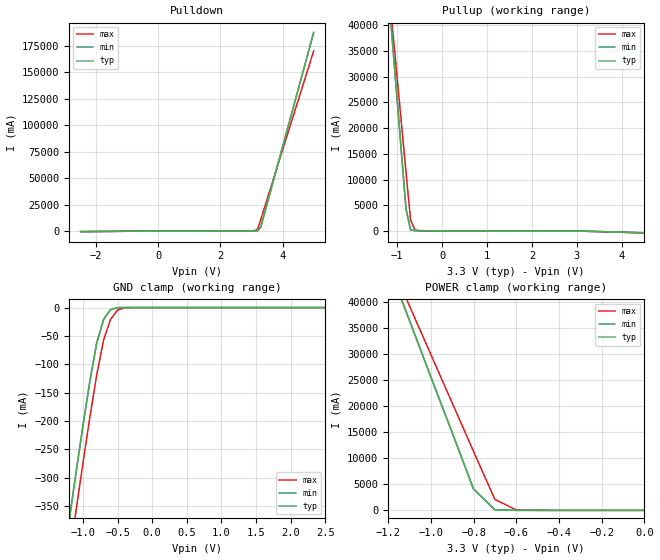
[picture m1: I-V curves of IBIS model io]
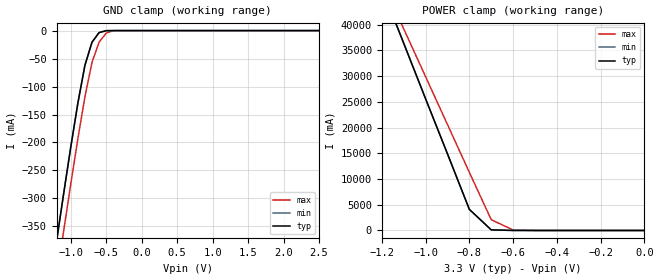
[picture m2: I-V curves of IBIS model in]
[IBIS Ver]   1.1
[File name]   m69737tq.ibs
[File Rev]   1.0
[Date]   4/7/98
[Source]   This file originated at Motorola FSRAM.
[Notes]
 1. This I/O model good for MCM69737 128Kx36 4Meg BurstRAM "F" and "P"
 versions (TQFP).
[Disclaimer]   Data is for modeling purposes only and is not guaranteed
[Component]   128Kx36 4M BurstRAM
[Manufacturer] Motorola
[Package]
|  RLC Data is subject to change after further study of package
|		typ		min		max
R_pkg		200m		150m		250m
L_pkg		5.5nH		4nH		7nH
C_pkg		2pF		1.5pF		2.5pF
[Pin]		signal_name	model_name	R_pin		L_pin		C_pin
1		DCc		io		NA		NA		NA
2		DCc		io		NA		NA		NA
3		DCc		io		NA		NA		NA
4		VDDQ		POWER		NA		NA		NA
5		VSS		GND		NA		NA		NA
6		DCc		io		NA		NA		NA
7		DCc		io		NA		NA		NA
8		DQc		io		NA		NA		NA
9		DQc		io		NA		NA		NA
10		VSS		GND		NA		NA		NA
11		VDDQ		POWER		NA		NA		NA
12		DQc		io		NA		NA		NA
13		DQc		io		NA		NA		NA
14		NC		NC		NA		NA		NA
15		VDD		POWER		NA		NA		NA
16		NC		NC		NA		NA		NA
17		VSS		GND		NA		NA		NA
18		DQd		io		NA		NA		NA
19		DQd	 	io		NA		NA		NA
20		VDDQ		POWER		NA		NA		NA
21		VSS		GND		NA		NA		NA
22		DQd		io		NA		NA		NA
23		DQd		io		NA		NA		NA
24		DQd		io		NA		NA		NA
25		DCd		NC		NA		NA		NA
26		VSS		GND		NA		NA		NA
27		VDDQ		POWER		NA		NA		NA
28		DCd		io		NA		NA		NA
29		DCd		io		NA		NA		NA
30		DCd		io		NA		NA		NA
31		LBO#		NC		NA		NA		NA
32		SA		in		NA		NA		NA
33		SA		in		NA		NA		NA
34		SA		in		NA		NA		NA
35		SA		in		NA		NA		NA
36		SA1		in		NA		NA		NA
37		SA0		in		NA		NA		NA
38		NC		NC		NA		NA		NA
39		NC		NC		NA		NA		NA
40		VSS		GND		NA		NA		NA
41		VDD		POWER		NA		NA		NA
42		NC		NC		NA		NA		NA
43		NC		NC		NA		NA		NA
44		SA		in		NA		NA		NA
45		SA		in		NA		NA		NA
46		SA		in		NA		NA		NA
47		SA		in		NA		NA		NA
48		SA		in		NA		NA		NA
49		SA		in		NA		NA		NA
50		SA		in		NA		NA		NA
51		DQa		io		NA		NA		NA
52		DQa		io		NA		NA		NA
53		DQa		io		NA		NA		NA
54		VDDQ		POWER		NA		NA		NA
55		VSS		GND		NA		NA		NA
56		DQa		io		NA		NA		NA
57		DQa		io		NA		NA		NA
58		DQa		io		NA		NA		NA
59		DQa		io		NA		NA		NA
60		VSS		GND		NA		NA		NA
61		VDDQ		POWER		NA		NA		NA
62		DQa		io		NA		NA		NA
63		DQa		io		NA		NA		NA
64		NC		NC		NA		NA		NA
65		VDD		POWER		NA		NA		NA
66		NC		NC		NA		NA		NA
67		VSS		GND		NA		NA		NA
68		DQb		io		NA		NA		NA
69		DQb		io		NA		NA		NA
70		VDDQ		POWER		NA		NA		NA
71		VSS		GND		NA		NA		NA
72		DQb		io		NA		NA		NA
73		DQb		io		NA		NA		NA
74		DQb		io		NA		NA		NA
75		DQb		io		NA		NA		NA
76		VSS		GND		NA		NA		NA
77		VDDQ		POWER		NA		NA		NA
78		DQb		io		NA		NA		NA
79		DQb		io		NA		NA		NA
80		DQb		io		NA		NA		NA
81		SA		in		NA		NA		NA
82		SA		in		NA		NA		NA
83		ADV		in		NA		NA		NA
84		ADSP		in		NA		NA		NA
85		ADSC		in		NA		NA		NA
86		G		in		NA		NA		NA
87		SW		in		NA		NA		NA
88		SGW		in		NA		NA		NA
89		K		in		NA		NA		NA
90		VSS		GND		NA		NA		NA
91		VDD		POWER		NA		NA		NA
92		SE3		in		NA		NA		NA
93		SBA		in		NA		NA		NA
94		SBB		in		NA		NA		NA
95		NC		NC		NA		NA		NA
96		NC		NC		NA		NA		NA
97		SE2		in		NA		NA		NA
98		SE1		in		NA		NA		NA
99		SA		in		NA		NA		NA
100		SA		in		NA		NA		NA
| Models and submodels in the file (2): io (I/O), in (Input)
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| BI-DIRECTIONAL I/O MODEL
[Model]   io
Model_type  I/O
Polarity   Non-Inverting
Enable   Active-Low
|signals  DQa, DQb, DQc, DQd
|Variable   typ   min   max
C_comp   7pF   NA   8pF
|Variable   typ   min   max
[Voltage range]   3.3   3.1  3.6
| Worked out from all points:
|   slope of the pulldown table from 0 to 0.495 V, typ, clamps not added: 19.4 ohm
|   slope of the pullup table from 0 to 0.495 V, typ, clamps not added: 18.1 ohm
|   GND clamp passes 1 mA (typ) near -0.52 V on its own axis
|   POWER clamp passes 1 mA (typ) near -0.53 V on its own axis
|Temp used   50C   100C   0C
|Variable   typ   min   max
|NOTE: All V/I tables should have at least 3 entries.
|   0.0 volts, 2*supply_voltage and -supply_voltage
[Pulldown]
|Voltage	Typical			Minimum		Maximum
-2.5V     -454.1mA   -454.2mA   -476.2mA
3V        59.2mA     68.8mA     53.1mA
3.1V      62.5mA     72.1mA     142.5mA
3.2V      178.6mA    188.2mA    2.1A
3.3V      4.2A       4.2A       11.3A
5V        187.4A     187.4A     170A
[Pullup]
|Voltage	Typical			Minimum		Maximum
-2.5V     187.5A     187.5A     170.1A
-1.2V     47.3A      47.3A      48.7A
-1.1V     36.5A      36.5A      39.3A
-1V       25.7A      25.7A      30A
-800mV    4.2A       4.2A       11.3A
-700mV    171.2mA    171.2mA    2.1A
-600mV    47.4mA     47.4mA     134.6mA
-500mV    36.6mA     36.6mA     38.2mA
3V        -50mA      -50mA      -52.9mA
5V        -507.3mA   -507.3mA   -528.3mA
[GND_clamp]
|Voltage	Typical			Minimum		Maximum
-2.5V     -1.5A      -1.5A      -1.6A
-1.2V     -377mA     -377mA     -444.1mA
-1.1V     -291.8mA   -291.8mA   -358.6mA
-1V       -208.8mA   -208.8mA   -274.8mA
-900mV    -130.2mA   -130.2mA   -193.9mA
-800mV    -62.1mA    -62.1mA    -118.6mA
-700mV    -20.7mA    -20.7mA    -56.6mA
-600mV    -3.6mA     -3.6mA     -20.8mA
-500mV    -153.5uA   -153.5uA   -4.4mA
-400mV    -4.3uA     -4.3uA     -310.1uA
2.5V      23.4pA     22.8pA     1.3nA
[POWER_clamp]
|Voltage	Typical		Minimum	Maximum
-2.5V     187.7A     187.5A     170.4A
-1.2V     47.2A      47.2A      48.6A
-1.1V     36.4A      36.4A      39.2A
-1V       25.6A      25.6A      29.9A
-800mV    4.1A       4.1A       11.3A
-700mV    119.3mA    119.3mA    2.1A
-600mV    3.3mA      3.3mA      93.5mA
0V        23.4pA     22.8pA     1.3nA
[Ramp]
|Variable   typ   min   max
dV/dt_r  1.089/0.21n   1.071/0.24n   1.11/0.188n
dV/dt_f  1.078/0.25n   1.023/0.309n	  1.12/0.193n
| STANDARD INPUT MODEL
[Model]   in
Model_type  Input
Polarity   Non-Inverting
|signals  /adsp, /adsc, /adv, /g, k, sa, /sbx, /se1, se2, /se3, /sgw, /sw
|Variable   typ   min   max
C_comp   7pF   NA   8pF
|Variable   typ   min   max
[Voltage range]   3.3   3.1  3.6
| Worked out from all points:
|   GND clamp passes 1 mA (typ) near -0.52 V on its own axis
|   POWER clamp passes 1 mA (typ) near -0.53 V on its own axis
|Temp used   50C   100C   0C
[GND_clamp]
|Voltage	Typical			Minimum		Maximum
-2.5V     -1.5A      -1.5A      -1.6A
-1.2V     -377mA     -377mA     -444.1mA
-1.1V     -291.8mA   -291.8mA   -358.6mA
-1V       -208.8mA   -208.8mA   -274.8mA
-900mV    -130.2mA   -130.2mA   -193.9mA
-800mV    -62.1mA    -62.1mA    -118.6mA
-700mV    -20.7mA    -20.7mA    -56.6mA
-600mV    -3.6mA     -3.6mA     -20.8mA
-500mV    -153.5uA   -153.5uA   -4.4mA
-400mV    -4.3uA     -4.3uA     -310.1uA
2.5V      23.4pA     22.8pA     1.3nA
[POWER_clamp]
|Voltage	Typical		Minimum	Maximum
-2.5V     187.7A     187.5A     170.4A
-1.2V     47.2A      47.2A      48.6A
-1.1V     36.4A      36.4A      39.2A
-1V       25.6A      25.6A      29.9A
-800mV    4.1A       4.1A       11.3A
-700mV    119.3mA    119.3mA    2.1A
-600mV    3.3mA      3.3mA      93.5mA
0V        23.4pA     22.8pA     1.3nA
